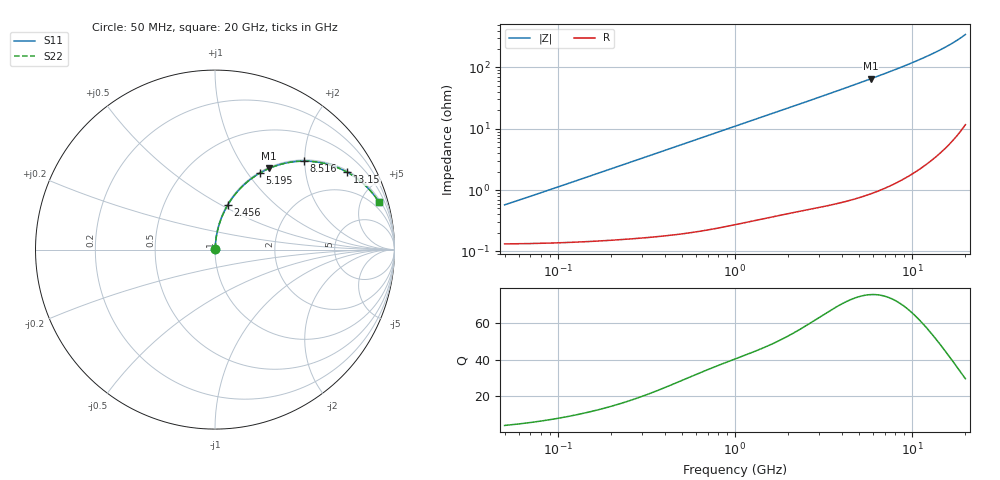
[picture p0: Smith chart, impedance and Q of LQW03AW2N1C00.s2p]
!Murata Part Number: LQW03AW2N1C00
!These Parameters are Measured in Series Mode Connection
!  o--[Z]--o
!Port1  Port2
!  o-------o
!Freq. Start=50[MHz] Stop=20[GHz], 401[Steps]
# Hz S RI R 50
!Freq.(Hz) S11(Real) S11(Imag) S21(Real) S21(Imag) S12(Real) S12(Imag) S22(Real) S22(Imag)
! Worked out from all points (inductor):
!   401 points, 50 MHz to 20 GHz, reference 50 ohm
!   read as one part in series: L = 1.77 nH near 51.52 MHz
!   highest Q = 75.3 at 5.856 GHz (marker M1), where L = 1.78 nH
!   S11 on the Smith chart (normalised r, x): 50 MHz: 1.00, +0.01; 2.456 GHz: 1.01, +0.54; 5.195 GHz: 1.02, +1.15; 8.516 GHz: 1.03, +1.97; 13.15 GHz: 1.06, +3.38; 20 GHz: 1.23, +6.89
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5e7  0.00135 0.00556  0.9986 -0.00556  0.9986 -0.00556  0.00135 0.00556
6.354076e7  0.00138 0.00706  0.9986 -0.00706  0.9986 -0.00706  0.00138 0.00706
1.364002e8  0.00165 0.0151  0.9983 -0.0151  0.9983 -0.0151  0.00165 0.0151
3.721004e8  0.00342 0.0408  0.9966 -0.0408  0.9966 -0.0408  0.00342 0.0408
6.285508e8  0.00683 0.0685  0.9932 -0.0685  0.9932 -0.0685  0.00683 0.0685
1e9  0.0145 0.1077  0.9855 -0.1077  0.9855 -0.1077  0.0145 0.1077
1.590961e9  0.0326 0.1674  0.9674 -0.1674  0.9674 -0.1674  0.0326 0.1674
2.456456e9  0.0707 0.2479  0.9293 -0.2479  0.9293 -0.2479  0.0707 0.2479
2.728004e9  0.0852 0.271  0.9148 -0.271  0.9148 -0.271  0.0852 0.271
3.265178e9  0.1168 0.3136  0.8832 -0.3136  0.8832 -0.3136  0.1168 0.3136
3.850025e9  0.1549 0.3547  0.8451 -0.3547  0.8451 -0.3547  0.1549 0.3547
4.472136e9  0.1986 0.3921  0.8014 -0.3921  0.8014 -0.3921  0.1986 0.3921
5.194772e9  0.2519 0.4274  0.7481 -0.4274  0.7481 -0.4274  0.2519 0.4274
5.856089e9  0.3017 0.4524  0.6983 -0.4524  0.6983 -0.4524  0.3017 0.4524
7.442007e9  0.419 0.4867  0.581 -0.4867  0.581 -0.4867  0.419 0.4867
8.516016e9  0.4931 0.4929  0.5069 -0.4929  0.5069 -0.4929  0.4931 0.4929
1.050288e10  0.6133 0.4792  0.3867 -0.4792  0.3867 -0.4792  0.6133 0.4792
1.166392e10  0.6726 0.4609  0.3274 -0.4609  0.3274 -0.4609  0.6726 0.4609
1.314879e10  0.7373 0.4308  0.2627 -0.4308  0.2627 -0.4308  0.7373 0.4308
1.621653e10  0.8375 0.3571  0.1625 -0.3571  0.1625 -0.3571  0.8375 0.3571
1.855685e10  0.8901 0.2984  0.1099 -0.2984  0.1099 -0.2984  0.8901 0.2984
2e10  0.9148 0.2627  0.0852 -0.2627  0.0852 -0.2627  0.9148 0.2627
